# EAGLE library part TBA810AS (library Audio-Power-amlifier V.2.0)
http://www.datasheetcatalog.com/datasheets_pdf/T/B/A/8/TBA810AS.shtml
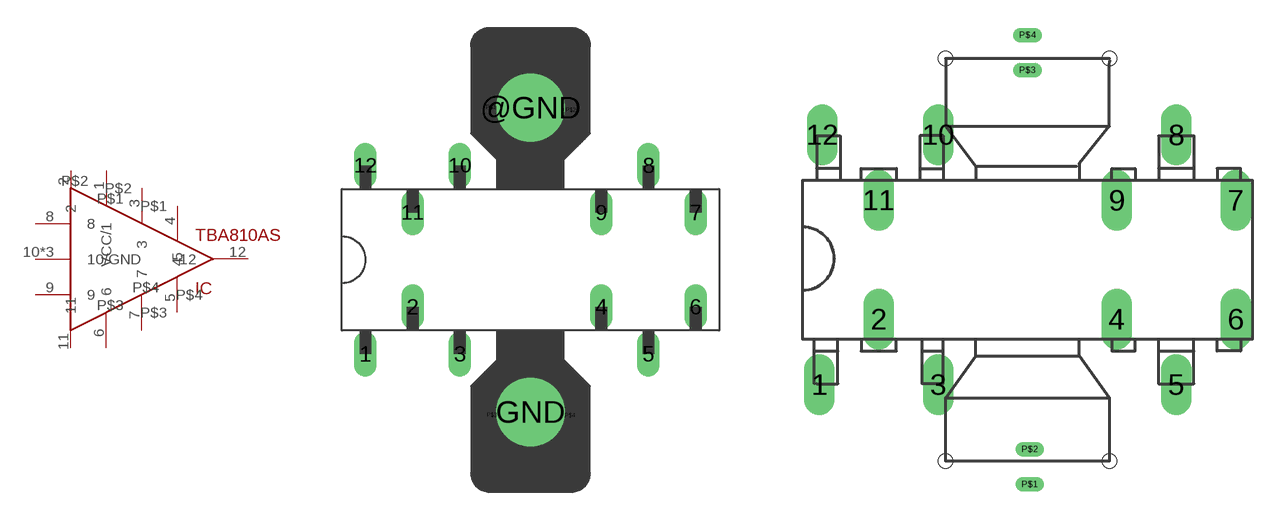
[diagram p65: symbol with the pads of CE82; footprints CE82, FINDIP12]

Designator prefix IC

## TBA810ASCB-155  [CE82]
1  VCC/1  pwr
2  2  nc
3  3
4  4
5  5
6  6
7  7
8  8  in
9  9  in
10  10/GND  pwr
11  11  nc
12  12  out
@GND  10/GND  pwr
GND  10/GND  pwr
P$1  P$1  pwr
P$2  P$2  pwr
P$3  P$3  pwr
P$4  P$4  pwr

## TBA810AS  [FINDIP12]
1  VCC/1  pwr
2  2  nc
3  3
4  4
5  5
6  6
7  7
8  8  in
9  9  in
10  10/GND  pwr
11  11  nc
12  12  out
P$1  P$1  pwr
P$2  P$2  pwr
P$3  P$3  pwr
P$4  P$4  pwr

## Footprint CE82 (pad centres in mm)
Package DIL 16 (CE83)
drill 0.7 long: 1 -8.89,-5.08; 2 -6.35,-2.54; 3 -3.81,-5.08; 4 3.81,-2.54; 5 6.35,-5.08; 6 8.89,-2.54; 7 8.89,2.54; 8 6.35,5.08; 9 3.81,2.54; 10 -3.81,5.08; 11 -6.35,2.54; 12 -8.89,5.08
drill 3.8: @GND 0,8.2; GND 0,-8.2
drill 0 pad 0.254: P$1 -2.12,8.22; P$2 2.17,8.07; P$3 -2.08,-8.37; P$4 2.12,-8.39

## Footprint FINDIP12 (pad centres in mm)
drill 0.8 long: 1 -8.89,-5.334; 2 -6.35,-2.54; 3 -3.81,-5.334; 4 3.81,-2.54; 5 6.35,-5.334; 6 8.89,-2.54; 7 8.89,2.54; 8 6.35,5.334; 9 3.81,2.54; 10 -3.81,5.334; 11 -6.35,2.54; 12 -8.763,5.334
drill 0 pad 0.61 long: P$1 0.1,-9.6; P$2 0.1,-8.1; P$3 0,8.1; P$4 0,9.6
hole 0.6 at -3.5,-8.6
hole 0.6 at 3.5,-8.6
hole 0.6 at 3.5,8.6
hole 0.6 at -3.5,8.6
